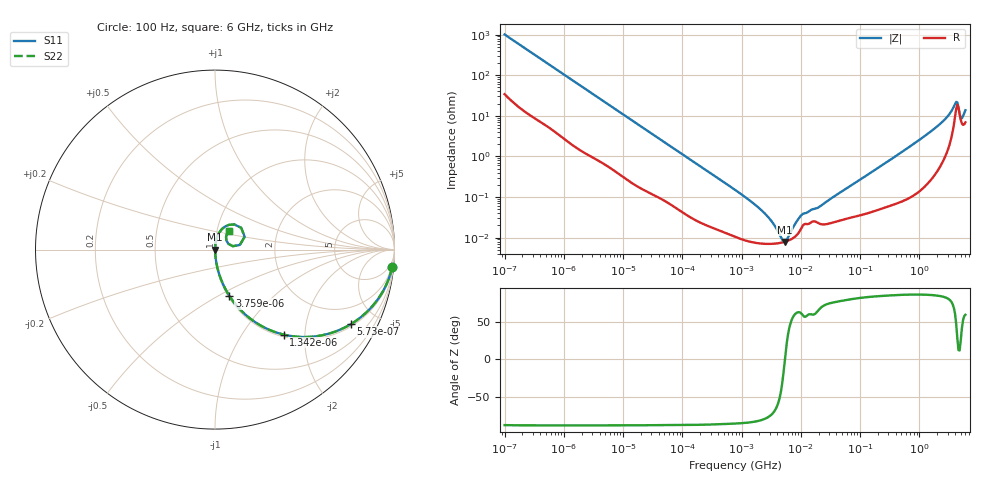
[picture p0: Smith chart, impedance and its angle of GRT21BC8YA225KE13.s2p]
!Murata Part Number: GRT21BC8YA225KE13
!These Parameters are Measured in Series Mode Connection
!Data Generated on Jun 19, 2026
!  o--ll--o
!Port1  Port2
!  o------o
!Operation Temp=25[degC], DC Bias Voltage=0[V]
!Freq. Start=100[Hz] Stop=6[GHz] 401[Steps]
# Hz S RI R 50
!Freq.(Hz) S11(Real) S11(Imag) S21(Real) S21(Imag) S12(Real) S12(Imag) S22(Real) S22(Imag)
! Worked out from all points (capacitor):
!   401 points, 100 Hz to 6 GHz, reference 50 ohm
!   read as one part in series: C = 1.57 uF near 109 Hz
!   lowest |Z| = 7.87 mohm at 5.312 MHz (marker M1)
!   series resonance near 5.39 MHz, so ESL is about 550 pH
!   S11 on the Smith chart (normalised r, x): 100 Hz: 2, -20; 573 Hz: 1.10, -3.61; 1.342 kHz: 1.04, -1.56; 3.759 kHz: 1.02, -0.57; 6 GHz: 1.14, +0.24
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100  0.987 -0.0975  0.013 0.0975  0.013 0.0975  0.987 -0.0975
280  0.9242 -0.2514  0.0758 0.2514  0.0758 0.2514  0.9242 -0.2514
573  0.759 -0.414  0.241 0.414  0.241 0.414  0.759 -0.414
1342  0.3822 -0.4734  0.6178 0.4734  0.6178 0.4734  0.3822 -0.4734
2008  0.222 -0.4031  0.778 0.4031  0.778 0.4031  0.222 -0.4031
3759  0.0805 -0.2584  0.9195 0.2584  0.9195 0.2584  0.0805 -0.2584
10527  0.0134 -0.1015  0.9866 0.1015  0.9866 0.1015  0.0134 -0.1015
40335  0.00172 -0.0275  0.9983 0.0275  0.9983 0.0275  0.00172 -0.0275
774597  0.000107 -0.0015  0.9999 0.0015  0.9999 0.0015  0.000107 -0.0015
2268635  7.1e-05 -0.000438  0.9999 0.000438  0.9999 0.000438  7.1e-05 -0.000438
3245845  7.03e-05 -0.000238  0.9999 0.000238  0.9999 0.000238  7.03e-05 -0.000238
4643984  7.48e-05 -6.76e-05  0.9999 6.76e-05  0.9999 6.76e-05  7.48e-05 -6.76e-05
5311619  7.84e-05 -6.6e-06  0.9999 6.6e-06  0.9999 6.6e-06  7.84e-05 -6.6e-06
6353432  8.61e-05 7.57e-05  0.9999 -7.57e-05  0.9999 -7.57e-05  8.61e-05 7.57e-05
9941735  0.000159 0.000303  0.9998 -0.000303  0.9998 -0.000303  0.000159 0.000303
1.555665e7  0.000246 0.00043  0.9998 -0.00043  0.9998 -0.00043  0.000246 0.00043
3.124326e8  0.00066 0.00795  0.9993 -0.00795  0.9993 -0.00795  0.00066 0.00795
1.95892e9  0.00685 0.0527  0.9932 -0.0527  0.9932 -0.0527  0.00685 0.0527
3.205649e9  0.0291 0.1027  0.9709 -0.1027  0.9709 -0.1027  0.0291 0.1027
4.009986e9  0.1081 0.14  0.8919 -0.14  0.8919 -0.14  0.1081 0.14
5.245841e9  0.0632 0.0516  0.9368 -0.0516  0.9368 -0.0516  0.0632 0.0516
6e9  0.076 0.1026  0.924 -0.1026  0.924 -0.1026  0.076 0.1026
